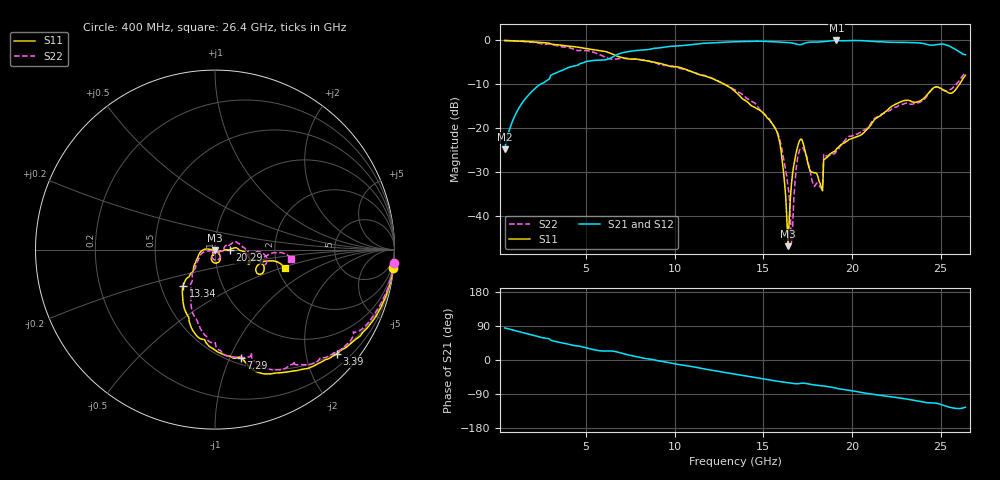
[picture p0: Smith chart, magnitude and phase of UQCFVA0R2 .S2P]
!  Part Number  UQCFVA0R2  Mounting Orientation: Horizontal
!  Description: Ultra Low ESR Microwave capacitors
!  Application: Coupling, Bypass, Tuning, DC Block
!  Filters, Matching
# GHZ S DB R 50
! Freq  |S11|  S11 Ph  |S21|  S21 Ph  |S12|  S12 Ph  |S22|  S22 Ph
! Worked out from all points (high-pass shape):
!   401 points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, 400 MHz to 26.4 GHz, reference 50 ohm
!   highest |S21| = 0.00 dB at 19.12 GHz (marker M1); lowest = -24.8 dB at 400 MHz (marker M2)
!   |S21| within 3 dB of the highest: 6.886 GHz to 26.22 GHz (19.33 GHz wide, 117 % of centre)
!   lowest |S11| = -46.8 dB at 16.39 GHz (marker M3), VSWR 1.01, Z = 49.8 - j0.398 ohm
!   |S11| at or under -10 dB: 12.82 GHz to 26.06 GHz (13.23 GHz wide, 68.1 % of centre)
!   |S22| runs from -46.1 to 0.0 dB; largest |S21 - S12| = 0.0027
!   S11 on the Smith chart (normalised r, x): 400 MHz: 0, -20; 3.39 GHz: 0.46, -2.65; 7.29 GHz: 0.56, -1.10; 13.34 GHz: 0.65, -0.28; 20.29 GHz: 1.18, -0.00; 26.4 GHz: 2.18, -0.54
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0.4  -0.02 -5.7  -24.76 84.8  -24.72 84.7  -0.01 -4.3
1.44  -0.18 -19.1  -13.93 71.9  -13.91 71.8  -0.21 -16.4
3.39  -0.97 -40.5  -7.20 47.7  -7.19 47.6  -1.20 -42.6
4.755  -1.69 -54.2  -5.17 34.8  -5.17 34.7  -2.29 -56.6
7.29  -4.12 -76.5  -2.60 14.4  -2.60 14.3  -4.09 -74.4
9.11  -5.19 -91.5  -1.70 -2.1  -1.71 -2.3  -5.42 -89.5
13.335  -11.37 -131.4  -0.30 -36.9  -0.31 -36.9  -11.09 -119.1
13.4  -11.60 -131.9  -0.28 -37.3  -0.29 -37.4  -11.24 -119.6
15.74  -20.53 -162.8  -0.32 -55.6  -0.34 -55.6  -20.49 -154.6
16  -25.13 177.1  -0.40 -57.3  -0.41 -57.4  -23.83 -168.1
16.39  -46.78 -119.3  -0.48 -59.8  -0.49 -59.8  -33.04 -165.1
16.52  -36.13 -42.9  -0.52 -60.8  -0.53 -60.8  -39.27 -156.2
16.65  -30.17 -44.8  -0.60 -61.8  -0.61 -61.8  -42.52 -48.4
17.04  -22.79 -73.4  -0.97 -62.1  -0.99 -62.0  -24.93 -64.1
17.755  -29.95 -104.6  -0.37 -65.1  -0.38 -65.0  -31.95 -115.4
18.21  -32.64 -125.3  -0.32 -67.6  -0.33 -67.6  -33.43 -107.9
18.535  -26.74 -6.7  -0.20 -69.5  -0.21 -69.4  -26.28 -4.2
19.12  -24.74 -0.2  0.00 -74.6  -0.01 -74.6  -25.20 15.0
20.29  -21.85 -1.2  -0.01 -83.7  -0.01 -83.6  -21.32 17.9
22.11  -15.41 -5.3  -0.40 -96.5  -0.40 -96.5  -15.96 4.8
25.49  -11.97 -25.7  -1.27 -124.5  -1.29 -124.4  -11.28 -10.4
26.4  -7.92 -15.0  -3.24 -124.6  -3.24 -124.6  -7.38 -7.0
